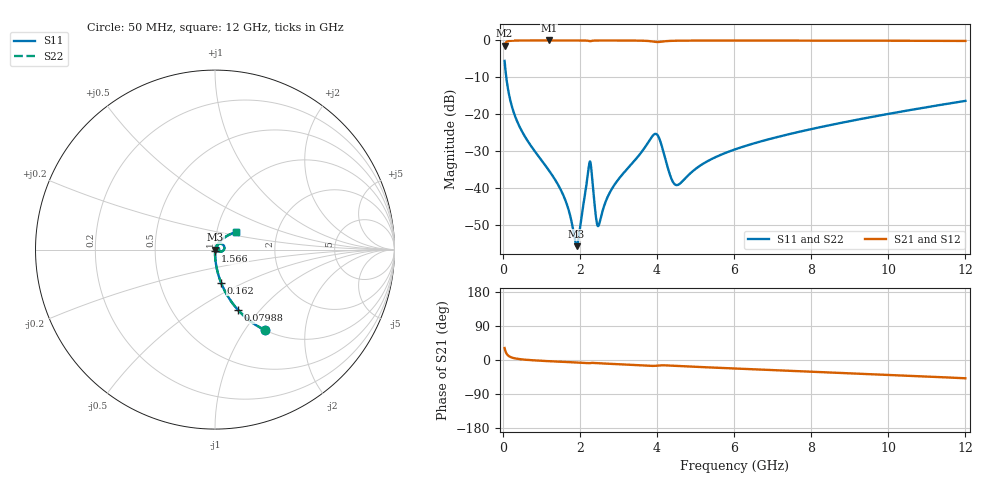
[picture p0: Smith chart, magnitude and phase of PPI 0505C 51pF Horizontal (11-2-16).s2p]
# MHz S MA R 50
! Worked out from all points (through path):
!   1601 points, 50 MHz to 12 GHz, reference 50 ohm
!   highest |S21| = -0.01 dB at 1.2 GHz (marker M1); lowest = -1.4 dB at 50 MHz (marker M2)
!   group delay of S21, straight-line fit = 11.8 ps
!   lowest |S11| = -55.8 dB at 1.917 GHz (marker M3), VSWR 1.00, Z = 50.2 - j0.0366 ohm
!   |S11| at or under -10 dB: 93.02 MHz to end of sweep
!   |S22| runs from -55.8 to -5.6 dB; largest |S21 - S12| = 0
!   S11 on the Smith chart (normalised r, x): 50 MHz: 1.00, -1.24; 79.88 MHz: 1.00, -0.78; 162 MHz: 1.00, -0.38; 1.566 GHz: 1.00, -0.02; 12 GHz: 1.23, +0.25
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50  0.5274 -58.3  0.8494 31.7  0.8494 31.7  0.5274 -58.3
79.875  0.3619 -69.0  0.9319 20.9  0.9319 20.9  0.3619 -69.0
162.0312  0.1872 -79.6  0.9819 10.2  0.9819 10.2  0.1872 -79.6
475.7188  0.06186 -87.4  0.9974 1.9  0.9974 1.9  0.06186 -87.4
1200.188  0.01726 -89.6  0.9987 -3.1  0.9987 -3.1  0.01726 -89.6
1566.156  0.008099 -86.1  0.9986 -4.9  0.9986 -4.9  0.008099 -86.1
1917.188  0.001625 -13.0  0.9983 -6.6  0.9983 -6.6  0.001625 -13.0
2044.156  0.004042 50.6  0.9977 -7.2  0.9977 -7.2  0.004042 50.6
2253.281  0.02237 15.9  0.9794 -8.3  0.9794 -8.3  0.02237 15.9
2305.562  0.01666 -31.6  0.9846 -7.5  0.9846 -7.5  0.01666 -31.6
2425.062  0.003797 -24.7  0.9962 -8.3  0.9962 -8.3  0.003797 -24.7
2484.812  0.003076 16.1  0.997 -8.6  0.997 -8.6  0.003076 16.1
2925.469  0.01157 68.0  0.9975 -10.7  0.9975 -10.7  0.01157 68.0
3888.938  0.05091 35.4  0.9669 -15.6  0.9669 -15.6  0.05091 35.4
4038.312  0.04972 -0.3  0.9515 -14.5  0.9515 -14.5  0.04972 -0.3
4359.469  0.01403 -12.6  0.9857 -14.9  0.9857 -14.9  0.01403 -12.6
4508.844  0.01093 16.5  0.9905 -15.7  0.9905 -15.7  0.01093 16.5
5210.906  0.0215 59.9  0.9953 -19.0  0.9953 -19.0  0.0215 59.9
6025  0.03333 61.9  0.9957 -22.4  0.9957 -22.4  0.03333 61.9
8019.156  0.06306 56.4  0.9942 -30.6  0.9942 -30.6  0.06306 56.4
10013.31  0.1012 48.7  0.9906 -39.2  0.9906 -39.2  0.1012 48.7
12000  0.1515 40.1  0.9835 -48.3  0.9835 -48.3  0.1515 40.1
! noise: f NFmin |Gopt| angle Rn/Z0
50  0.0003857  0.8636  0.5562  0.0006065
1372  0.003999  0.6751  4.77  0.00237
2701  0.007702  0.6699  9.229  0.004458
4031  0.04483  0.904  13.77  0.1009
5360  0.01453  0.6591  18.12  0.007947
6682  0.01485  0.602  22.3  0.006643
8012  0.01645  0.5796  26.42  0.006772
9341  0.01835  0.5688  30.42  0.007199
1.067e+04  0.02042  0.5644  34.3  0.007767
1.2e+04  0.02264  0.5645  38.05  0.008443
